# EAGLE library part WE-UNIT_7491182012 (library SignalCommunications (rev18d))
WE-UNIT Off-Line Transformer Characteristics Nominal input voltage: 125–375 VDC (85–265 VAC) Output power 3 W and 9 W Operating temperature: –40 °C to +125 °C Clearance and creepage distance 6 mm min. Insulation test voltage: 4 kVAC, 1 Minute Design compliant to EN 61558-2-16: reinforced insulation; except 749 118 10 xx: Basic insulation Applications Designed for Tiny Switch ICs from Power Integration and NCP101x or 105x of ON Semiconductor For SMPS with universal input from 85 VAC up to 265 VAC Details see: http://katalog.we-online.de/en/pbs/WE-UNIT?m Updated by Dan Xu 2014-07-11 2014 (C) Wurth Elektronik
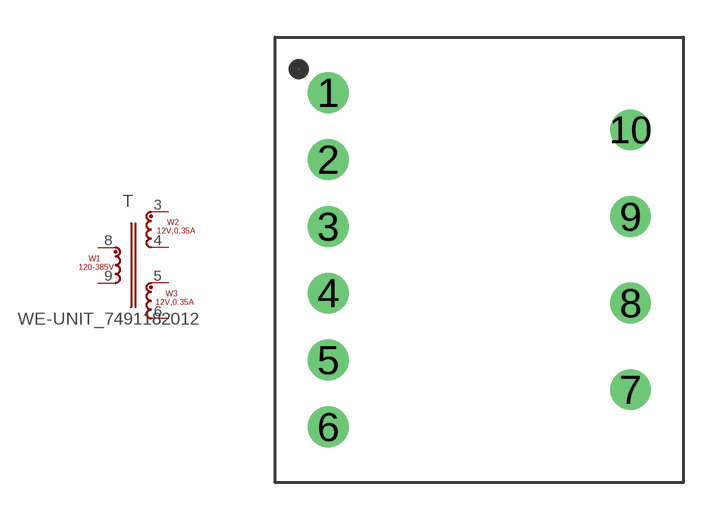
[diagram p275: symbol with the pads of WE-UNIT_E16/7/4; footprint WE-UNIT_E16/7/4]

Designator prefix T

## WE-UNIT_7491182012  [WE-UNIT_E16/7/4]
3  2  pas
4  3  pas
5  4  pas
6  5  pas
8  1  pas
9  6  pas

## Footprint WE-UNIT_E16/7/4 (pad centres in mm)
Transformer, E16/7/4 THT Vertikal 10 Pin
drill 1.1: 1 -6.1,6.75; 2 -6.1,4.05; 3 -6.1,1.35; 4 -6.1,-1.35; 5 -6.1,-4.05; 6 -6.1,-6.75; 7 6.1,-5.25; 8 6.1,-1.75; 9 6.1,1.75; 10 6.1,5.25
